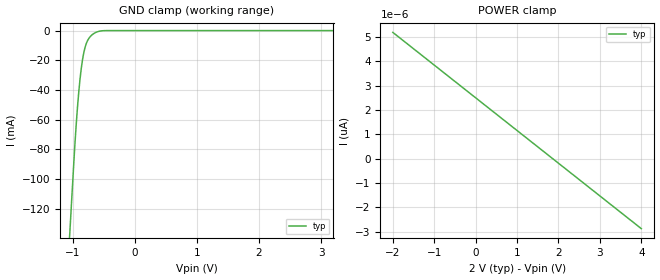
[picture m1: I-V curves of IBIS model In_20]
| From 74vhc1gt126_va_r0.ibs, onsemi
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|//////////////////////////////////////////////////////////////////////////////
|//////////////////////////////////////////////////////////////////////////////
[Model]  In_20
Model_type Input
Vinh =  1.00
Vinl =  0.28
|  variable   typ   min   max
C_comp   2.6pF   2.6pF   2.6pF
|//////////////////////////////////////////////////////////////////////////////
[Temperature Range]   25   125   -55
|//////////////////////////////////////////////////////////////////////////////
[Voltage Range]   2.00V   NA   NA
|//////////////////////////////////////////////////////////////////////////////
[POWER Clamp Reference] 2.00V   NA   NA
|//////////////////////////////////////////////////////////////////////////////
[GND Clamp Reference]   0V   NA   NA
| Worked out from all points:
|   GND clamp passes 1 mA (typ) near -0.61 V on its own axis
|//////////////////////////////////////////////////////////////////////////////
[GND Clamp]
|   Voltage   I(typ)   I(min)   I(max)
-2V       -836.7mA   NA         NA
-1.06V    -147.5mA   NA         NA
-1.03V    -125.5mA   NA         NA
-980mV    -88.84mA   NA         NA
-940mV    -62.39mA   NA         NA
-900mV    -41.15mA   NA         NA
-860mV    -25.44mA   NA         NA
-820mV    -14.98mA   NA         NA
-780mV    -8.793mA   NA         NA
-640mV    -1.545mA   NA         NA
-440mV    -9.08uA    NA         NA
4V        5.18pA     NA         NA
|//////////////////////////////////////////////////////////////////////////////
[POWER Clamp]
|   Voltage   I(typ)   I(min)   I(max)
-2V       5.18pA     NA         NA
0V        2.495pA    NA         NA
2V        -190.1fA   NA         NA
4V        -2.875pA   NA         NA
